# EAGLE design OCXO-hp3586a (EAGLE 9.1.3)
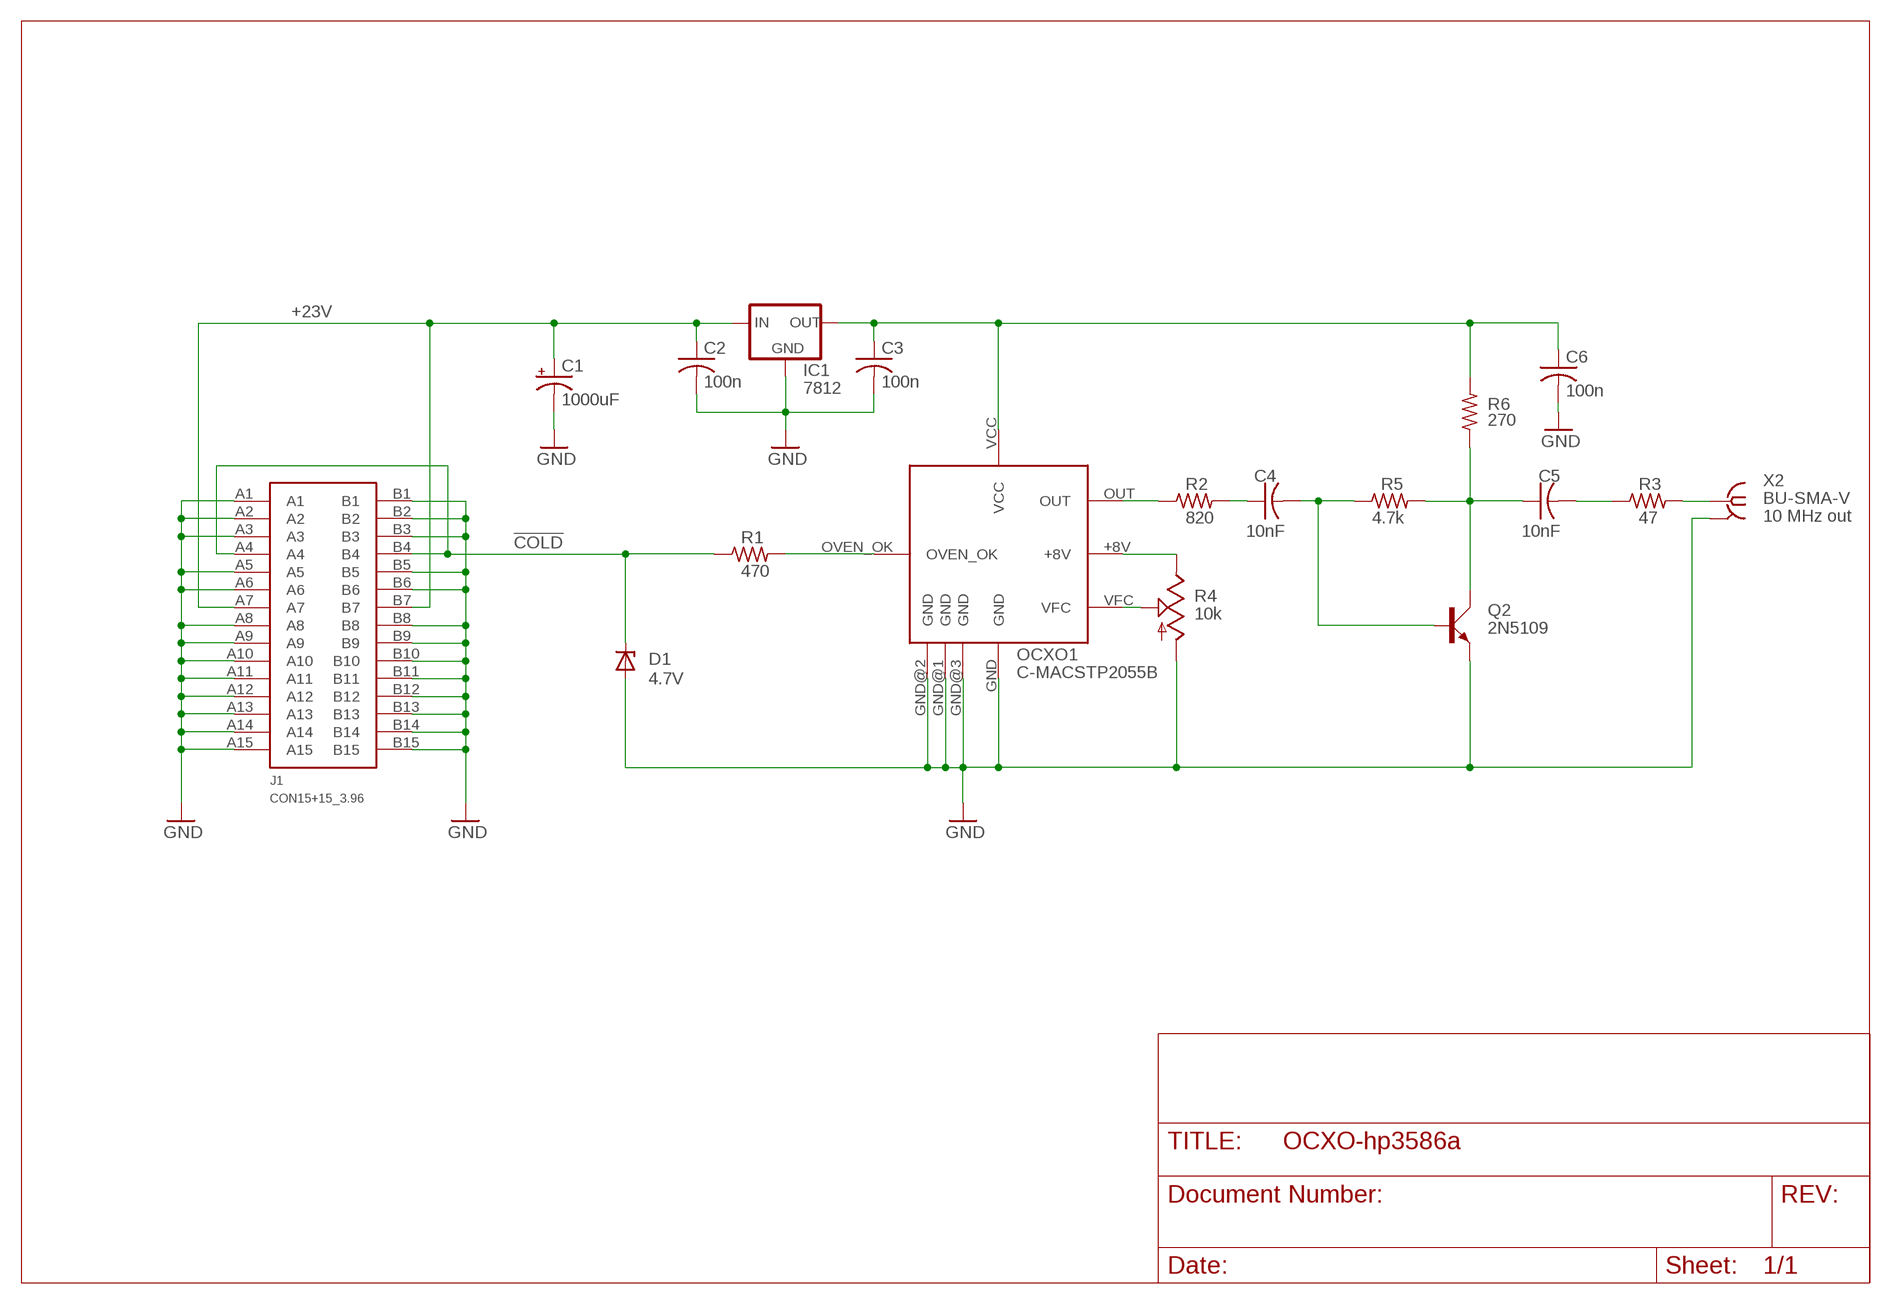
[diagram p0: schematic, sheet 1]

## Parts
C1  1000uF  CPOL-USE5-8.5  [E5-8,5]
C2  100n  C-US050-025X075  [C050-025X075]
C3  100n  C-US050-025X075  [C050-025X075]
C4  10nF  C-US050-024X044  [C050-024X044]
C5  10nF  C-US050-024X044  [C050-024X044]
C6  100n  C-US050-025X075  [C050-025X075]
D1  4.7V  ZENER-DIODEDO34-7  [DO34Z7]
IC1  7812  78XXL  [78XXL]
J1  CON15+15_3.96  [15+15_CARDEDGE_CONNECTOR_3.96MM]
OCXO1  C-MACSTP2055B  [CMAC-OCXO]
Q2  2N5109  TRANSISTOR-SMALL-SIGNAL_2N5109  [TRANSISTOR-SMALL-SIGNAL_TO5A]
R1  470  R-US_0207/10  [0207/10]
R2  820  R-US_0207/10  [0207/10]
R3  47  R-US_0207/10  [0207/10]
R4  10k  TRIM_US-S43P  [SP19L]
R5  4.7k  R-US_0207/10  [0207/10]
R6  270  R-US_0207/10  [0207/10]
X2  BU-SMA-V  [BU-SMA-V]

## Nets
!COLD: D1.C J1.A4 J1.B4 R1.1
+12V: C3.1 C6.1 IC1.OUT OCXO1.VCC R6.2
+23V: C1.+ C2.1 IC1.IN J1.A7 J1.B7
GND: C1.- C2.2 C3.2 C6.2 D1.A IC1.GND J1.A1 J1.A2 J1.A3 J1.A5 J1.A6 J1.A8 J1.A9 J1.A10 J1.A11 J1.A12 J1.A13 J1.A14 J1.A15 J1.B1 J1.B2 J1.B3 J1.B5 J1.B6 J1.B8 J1.B9 J1.B10 J1.B11 J1.B12 J1.B13 J1.B14 J1.B15 OCXO1.GND OCXO1.GND@1(GND) OCXO1.GND@2(GND) OCXO1.GND@3(GND) Q2.E R4.A X2.2 X2.3 X2.4 X2.5
N$1: OCXO1.OUT R2.1
N$2: R3.2 X2.1
N$3: OCXO1.VFC R4.S
N$4: OCXO1.+8V R4.E
N$5: C4.1 R2.2
N$6: C5.2 R3.1
N$7: OCXO1.OVEN_OK R1.2
N$8: C5.1 Q2.C R5.2 R6.1
N$9: C4.2 Q2.B R5.1

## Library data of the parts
C1 = rcl:CPOL-US: POLARIZED CAPACITOR, American symbol
C2-C6 = rcl:C-US: CAPACITOR, American symbol
D1 = diode:ZENER-DIODE: Z-Diode
IC1 = v-reg:78XXL: VOLTAGE REGULATOR
J1 = edgeconn15+15:CON15+15_3.96
OCXO1 = i1epj:C-MACSTP2055B
Q2 = OCXO-hp3586a:TRANSISTOR-SMALL-SIGNAL_2N5109: NPN TRANSISTOR
R1-R3 R5 R6 = rcl:R-US_: RESISTOR, American symbol
R4 = pot:TRIM_US-: POTENTIOMETER
X2 = con-coax:BU-SMA-V: FEMALE SMA CONNECTOR; INFO: 10 MHz out; OC_FARNELL: unknown; OC_NEWARK: unknown

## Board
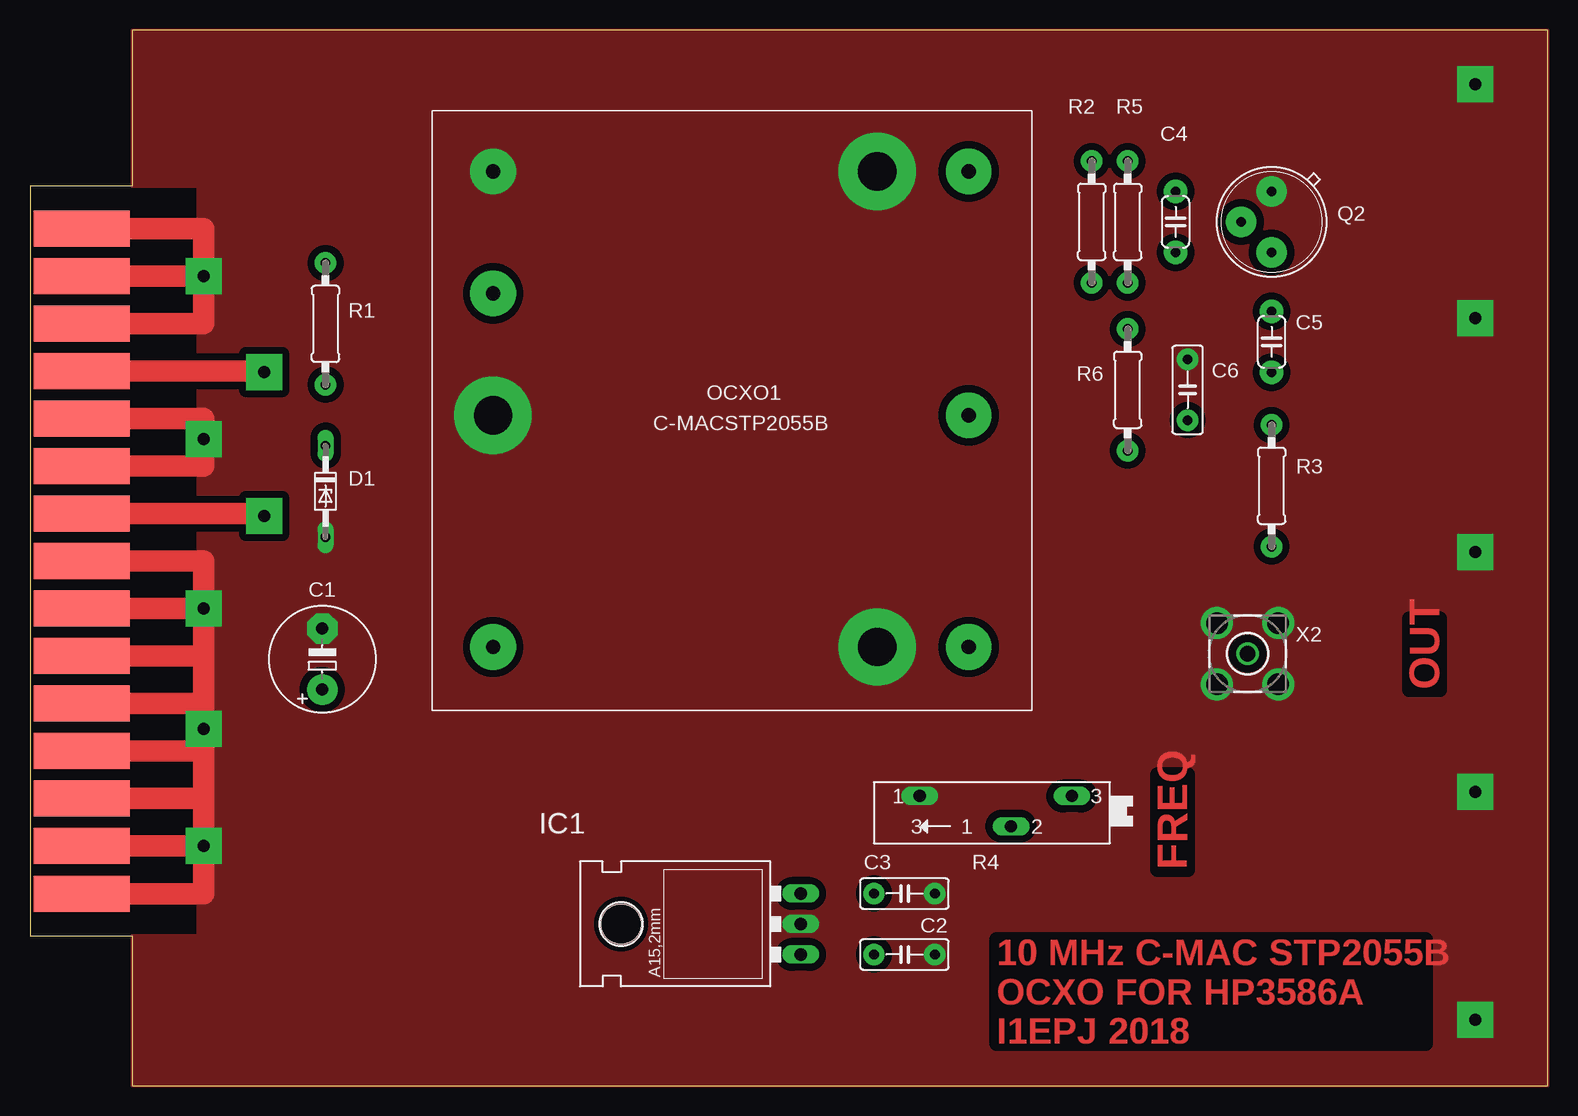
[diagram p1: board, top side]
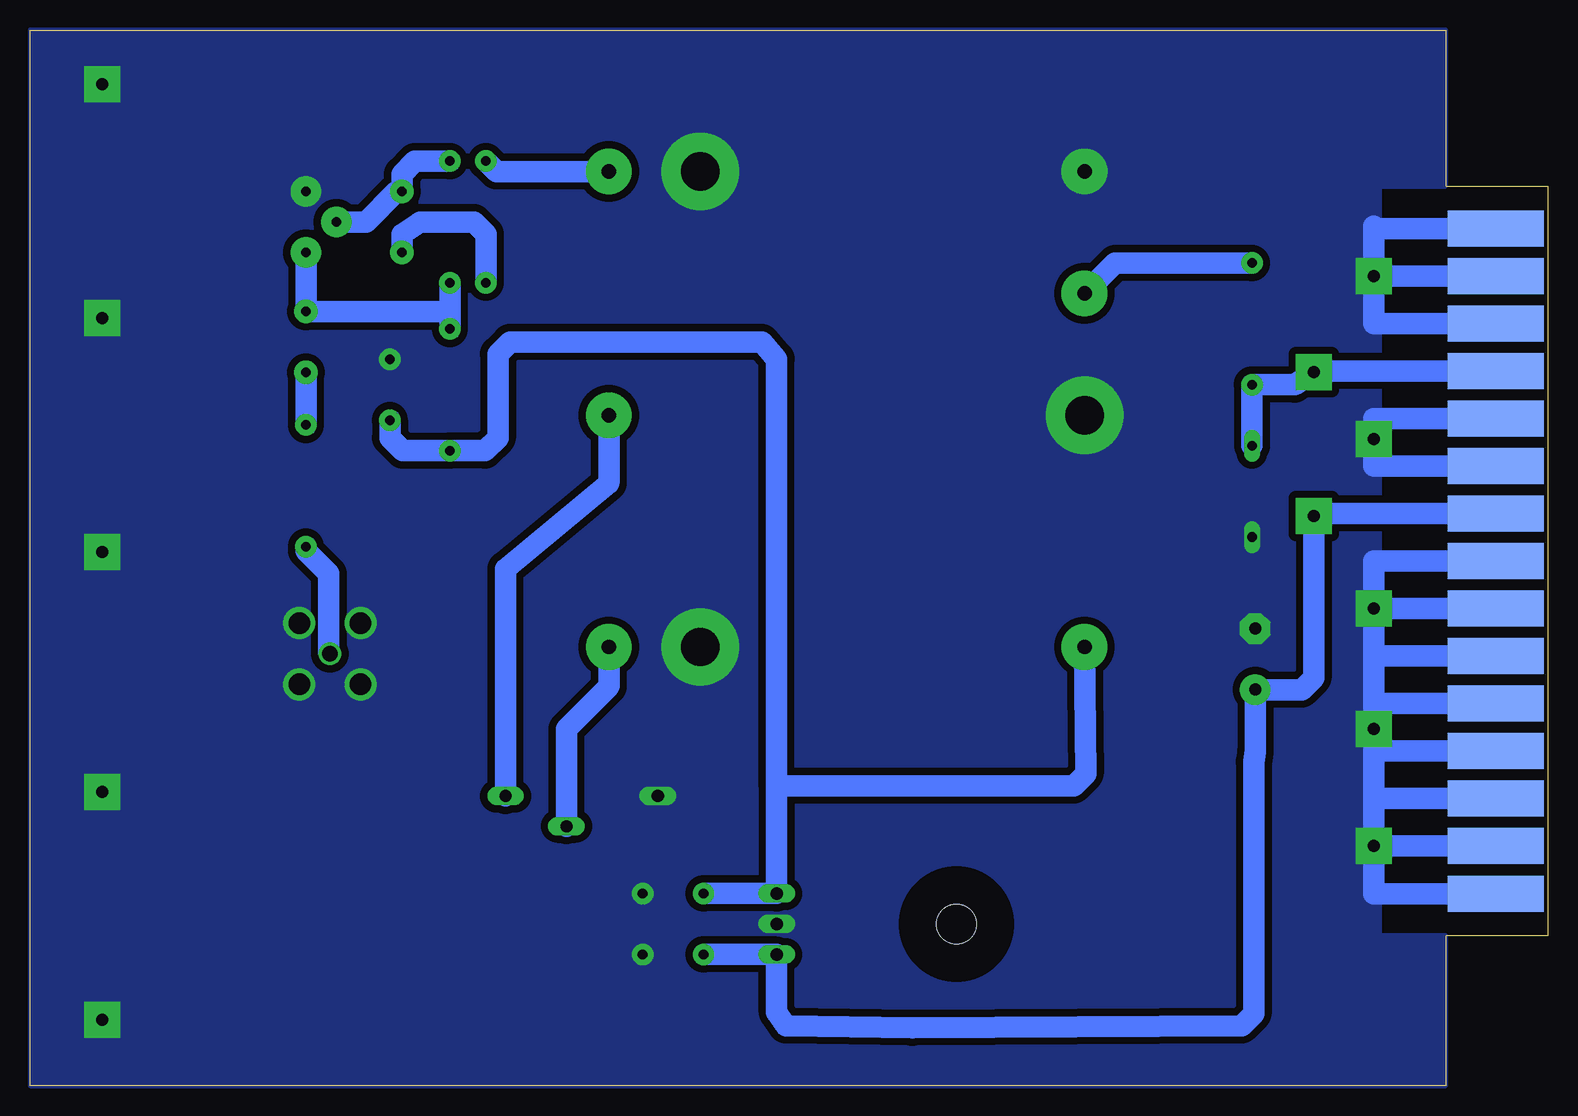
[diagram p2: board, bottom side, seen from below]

Size 126.5 x 88 mm. Coordinates in mm from the lower left corner, seen from the top.
Outline: 8.5,0 126.5,0 126.5,88 8.5,88 8.5,75 0,75 0,12.5 8.5,12.5 8.5,0
Copper layers (1*16): Top 0.035mm / dielectric 1.5mm / Bottom 0.035mm
Design rules "default *": minimum track width 10mil, minimum drill 24mil, track to track 8mil, track to pad 8mil, pad to pad 8mil, via to via 8mil, smd to smd 8mil, copper to edge 0mil, drill to drill 8mil, minimum pad ring 10mil, minimum via ring 8mil, stop-mask expansion 4mil, vias tented up to drill 0mil, thermal gap 0mil

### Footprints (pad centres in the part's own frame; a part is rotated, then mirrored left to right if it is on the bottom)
E5-8,5 = drill 1.016 pad 2.54: + -2.54,0 | drill 1.016 pad 2.54 octagon: - 2.54,0
C050-025X075 = drill 0.813 pad 1.778: 1 -2.54,0; 2 2.54,0
C050-024X044 = drill 0.813 pad 1.93: 1 -2.54,0; 2 2.54,0
DO34Z7 = drill 0.813 long: A 3.81,0; C -3.81,0
78XXL = drill 1.016 long: GND 0,-3.81; IN -2.54,-3.81; OUT 2.54,-3.81 | hole 3.302: 0,11.176
15+15_CARDEDGE_CONNECTOR_3.96MM = smd 3 x 8: A1 -27.72,0; A2 -23.76,0; A3 -19.8,0; A4 -15.84,0; A5 -11.88,0; A6 -7.92,0; A7 -3.96,0; A8 0,0; A9 3.96,0; A10 7.92,0; A11 11.88,0; A12 15.84,0; A13 19.8,0; A14 23.76,0; A15 27.72,0 | smd 3 x 8 bottom: B1 -27.72,0; B2 -23.76,0; B3 -19.8,0; B4 -15.84,0; B5 -11.88,0; B6 -7.92,0; B7 -3.96,0; B8 0,0; B9 3.96,0; B10 7.92,0; B11 11.88,0; B12 15.84,0; B13 19.8,0; B14 23.76,0; B15 27.72,0
CMAC-OCXO = drill 1.2 pad 3.81: +8V 25.4,44.72; GND 5.08,5.08; OUT 5.08,44.72; OVEN_OK 15.24,5.08; VCC 44.72,5.08; VFC 44.72,44.72 | drill 3.2 pad 6.452: GND@1 5.08,37.1; GND@2 44.72,37.1; GND@3 25.4,5.08
TRANSISTOR-SMALL-SIGNAL_TO5A = drill 0.813 pad 2.54: B 2.54,0; C 0,2.54; E 0,-2.54
0207/10 = drill 0.813 pad 1.778: 1 -5.08,0; 2 5.08,0
SP19L = drill 1.016 long: A 5.715,-1.27; E -6.985,-1.27; S -1.905,1.27
BU-SMA-V = drill 1.27: 1 0,0 | drill 1.778: 2 -2.55,2.55; 3 2.55,2.55; 4 2.55,-2.55; 5 -2.55,-2.55

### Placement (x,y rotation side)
C1  24.36,35.56 90 top
C2  72.89,10.92 0 top
C3  72.89,16 0 top
C4  95.5,72 90 top
C5  103.5,62 270 top
C6  96.5,58 90 top
D1  24.63,49.53 270 top
IC1  60.44,13.46 90 top
J1  4.31,43.72 270 top
OCXO1  33.52,81.28 270 top
Q2  103.5,72 180 top
R1  24.63,63.5 90 top
R2  88.5,72 270 top
R3  103.5,50 270 top
R4  79.88,22.88 180 top
R5  91.5,72 270 top
R6  91.5,58 270 top
X2  101.5,36 0 top

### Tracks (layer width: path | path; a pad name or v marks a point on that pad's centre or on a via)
!COLD  (via drill 1 pad 3)
  Top 1.8: J1.B4 18.94,59.56 v19.5,59.5
  Bottom 1.8: D1.C R1.1 21.08,58.42 v19.5,59.5 18.94,59.56 J1.B4
+12V
  Bottom 1.8: C3.1 IC1.OUT 64.25,24.89 | OCXO1.VCC 38.5,26 39.5,25 63.5,25 64.25,24.89 | C6.1 96.5,54 95.42,52.92 R6.2 88.58,52.92 87.5,54 87.5,61 86.5,62 65.5,62 64.25,60.58 64.25,24.89
+23V  (via drill 1 pad 3)
  Top 1.8: J1.B7 19.32,47.68 v19.5,47.5
  Bottom 1.8: C2.1 IC1.IN 64.25,6.1 63.5,5 52.95,4.81 25.5,5 24.5,6 24.5,27 24.36,27.86 C1.+ 24.34,33 20.5,33 19.5,34 v19.5,47.5 19.32,47.68 J1.B7
GND  (via drill 1 pad 3)
  Top 1.8: J1.B15 14.47,16 v14.47,19.96 | J1.B13 14.47,23.92 | 14.47,23.92 v14.47,19.96 | J1.B12 14.47,27.88 | 14.47,27.88 14.47,23.92 | J1.B11 14.47,31.84 | 14.47,31.84 v14.47,29.75 14.47,27.88 | J1.B10 14.47,35.8 | 14.47,35.8 14.47,31.84 | v14.47,39.76 14.47,35.8 | J1.B8 14.47,43.72 v14.47,39.76 | J1.B6 14.47,51.64 v14.47,53.88 14.47,55.6 J1.B5 | J1.B1 14.47,71.44 v14.47,67.48 | J1.B3 14.47,63.52 v14.47,67.48 | J1.B2 v14.47,67.48 | J1.B9 v14.47,39.76 | J1.B14 v14.47,19.96
  Bottom 1.8: J1.B1 14.47,71.44 | 14.47,71.44 14.47,71.66 | J1.B2 v14.47,67.48 | v14.47,67.48 14.47,71.44 | J1.B3 14.47,63.52 v14.47,67.48 | J1.B5 14.47,55.6 v14.47,53.88 14.47,51.64 J1.B6 | J1.B8 14.47,43.72 v14.47,39.76 | v14.47,39.76 14.47,35.8 | 14.47,35.8 v14.47,29.75 | J1.B9 v14.47,39.76 | J1.B10 14.47,35.8 | J1.B11 14.47,31.84 v14.47,29.75 | J1.B12 14.47,27.88 | 14.47,27.88 v14.47,29.75 | J1.B13 14.47,23.92 | 14.47,23.92 14.47,27.88 | J1.B14 v14.47,19.96 | v14.47,19.96 14.47,23.92 | J1.B15 14.47,16 v14.47,19.96
  other vias: 120.47,83.48 120.47,44.48 120.47,5.48 120.47,63.98 120.47,24.48
  pour Bottom (isolate 0.61, no thermals): 8.5,88 126.5,88 126.5,0 8.5,0 8.5,12.5 14,12.5 14,75 8.5,75
  pour Top (isolate 0.61): 8.5,88 8.5,75 14,75 14,12.5 8.5,12.5 8.5,0 126.5,0 126.5,88
N$1
  Bottom 1.8: OCXO1.OUT 87.62,76.2 R2.1
N$2
  Bottom 1.8: R3.2 103.5,44.58 101.59,42.67 101.59,36.09 X2.1
N$3
  Bottom 1.8: R4.S 81.78,29.72 78.26,33.24 78.24,33.32 OCXO1.VFC
N$4
  Bottom 1.8: R4.E 86.86,43.08 78.27,50.19 78.24,50.37 OCXO1.+8V
N$5
  Bottom 1.8: R2.2 88.5,71 89.5,72 93.96,72 95.5,71 C4.1
N$6
  Bottom 1.8: R3.1 C5.2
N$7
  Bottom 1.8: R1.2 36.06,68.58 OCXO1.OVEN_OK
N$8
  Bottom 1.8: R6.1 91.5,65 | 91.5,65 R5.2 | 91.5,65 91.96,64.54 C5.1 Q2.C
N$9
  Bottom 1.8: R5.1 94.42,77.08 95.5,76 C4.2 95.96,74.54 98.5,72 Q2.B

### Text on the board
Top: OUT | FREQ | 10 MHz C-MAC STP2055B / OCXO FOR HP3586A / I1EPJ 2018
